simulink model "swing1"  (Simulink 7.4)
settings: Solver=ode45  StartTime=0.0  StopTime=10.0  MaxStep=0.01  RelTol=1e-3
StartFcn:
  | close all
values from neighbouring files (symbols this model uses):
  D = str2num(get(h,'string'))    [acttrcalc1.m]
  f = input('Frequency [default = 1.0] =')    [Actac.m]    (also in alternator.m = getframe(gcf); brushlessdcB.m = getframe(gca); brushlessdcnew.m = getframe(gca); calc0.m = f+dfa*ti/6)
  H = 0.60    (= 0.6)    [IMabc2.m]    (also in IMcur0.m = 0.3; imdef0vec.m = 0.3; imdef1vec.m = 0.3; imdef2vec.m = 0.3)
  V = [Vas 0 0].'    [Actac.m]    (also in acttrcalc1.m = str2num(get(h,'string')); im3d.m = eval(get(hVs,'String')); IMabc2.m = [vas vbs vcs 0 0 0]'; IMabcf0.m = [vas vbs vcs 0 0 0]')
undefined symbols (not defined in the file or in its folder): Pm, t0, Tc, Xafter, Xbefore, Xduring

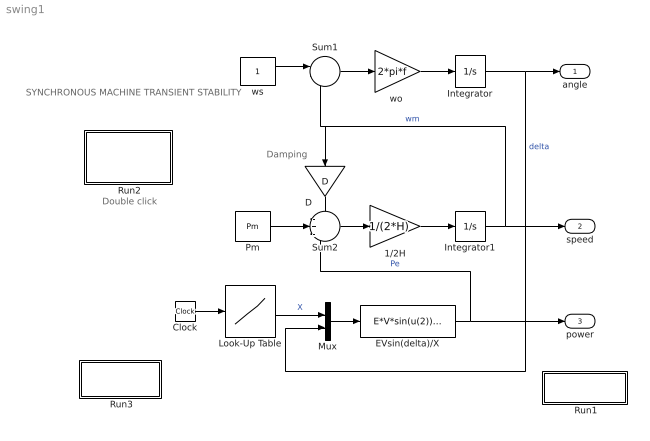
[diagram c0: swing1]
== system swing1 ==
  note: SYNCHRONOUS MACHINE TRANSIENT STABILITY
  note: Damping
  note: Double click
  " Run1" : Subsystem
  " Run2" : Subsystem
  " Run3" : Subsystem
  1/2H : Gain  Gain=1/(2*H)  ParameterDataType=sfix(16)  ParameterScaling=2^0  OutDataType=sfix(16)  OutScaling=2^0
  Clock : Clock
  D : Gain  Gain=D  ParameterDataType=sfix(16)  ParameterScaling=2^0  OutDataType=sfix(16)  OutScaling=2^0
  EVsin(delta)/X : Fcn  Expr=E*V*sin(u(2))/u(1)
  Integrator : Integrator
  Integrator1 : Integrator
  Look-Up Table : Lookup  InputValues=[0 t0 t0 t0+Tc t0+Tc 4]  Table=[Xbefore Xbefore Xduring Xduring Xafter Xafter]  OutDataType=sfix(16)  OutScaling=2^0
  Mux : Mux  Inputs=2
  Pm : Constant  Value=Pm  OutDataType=sfix(16)  OutScaling=2^0
  Sum1 : Sum  Inputs=|-+  OutDataType=sfix(16)  OutScaling=2^0
  Sum2 : Sum  Inputs=-+-  OutDataType=sfix(16)  OutScaling=2^0
  "wo " : Gain  Gain=2*pi*f  ParameterDataType=sfix(16)  ParameterScaling=2^0  OutDataType=sfix(16)  OutScaling=2^0
  ws : Constant  OutDataType=sfix(16)  OutScaling=2^0
  angle : Outport
  speed : Outport  Port=2
  power : Outport  Port=3
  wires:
  ws/1 -> Sum1/1
  Integrator/1 -> Mux/2, angle/1  "delta"
  Sum1/1 -> "wo "/1
  Mux/1 -> EVsin(delta)/X/1
  Sum2/1 -> 1/2H/1
  1/2H/1 -> Integrator1/1
  Integrator1/1 -> speed/1, Sum1/2, D/1  "wm"
  Pm/1 -> Sum2/2
  D/1 -> Sum2/1
  "wo "/1 -> Integrator/1
  EVsin(delta)/X/1 -> power/1, Sum2/3  "Pe"
  Clock/1 -> Look-Up Table/1
  Look-Up Table/1 -> Mux/1  "X"

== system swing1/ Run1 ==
  note: This demo simulates the transient stability problem in a single machine connected to an infinite bus. A sudden disturbance occurs which modifies the electrical output Pe while the mechanical input Pm remains constant. Swings curves are generated for specified clearing times Tc. Power-angle curves are also exhibited.
  note: Double click the block to enter the parameters and initial conditions and run the simulation

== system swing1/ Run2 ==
  note: This demo simulates the transient stability problem in a single machine connected to an infinite bus. A sudden disturbance occurs which modifies the electrical output Pe while the mechanical input Pm remains constant. Swings curves are generated for specified clearing times Tc. Power-angle curves are also exhibited.
  note: Double click the block to enter the parameters and initial conditions and run the simulation

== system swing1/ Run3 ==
  note: Double click the block to enter the parameters and initial conditions and run the simulation
  note: This demo simulates the transient stability problem in a single machine connected to an infinite bus. A sudden disturbance occurs which modifies the electrical output Pe while the mechanical input Pm remains constant. Swings curves are generated for specified clearing times Tc. Power-angle curves are also exhibited.
